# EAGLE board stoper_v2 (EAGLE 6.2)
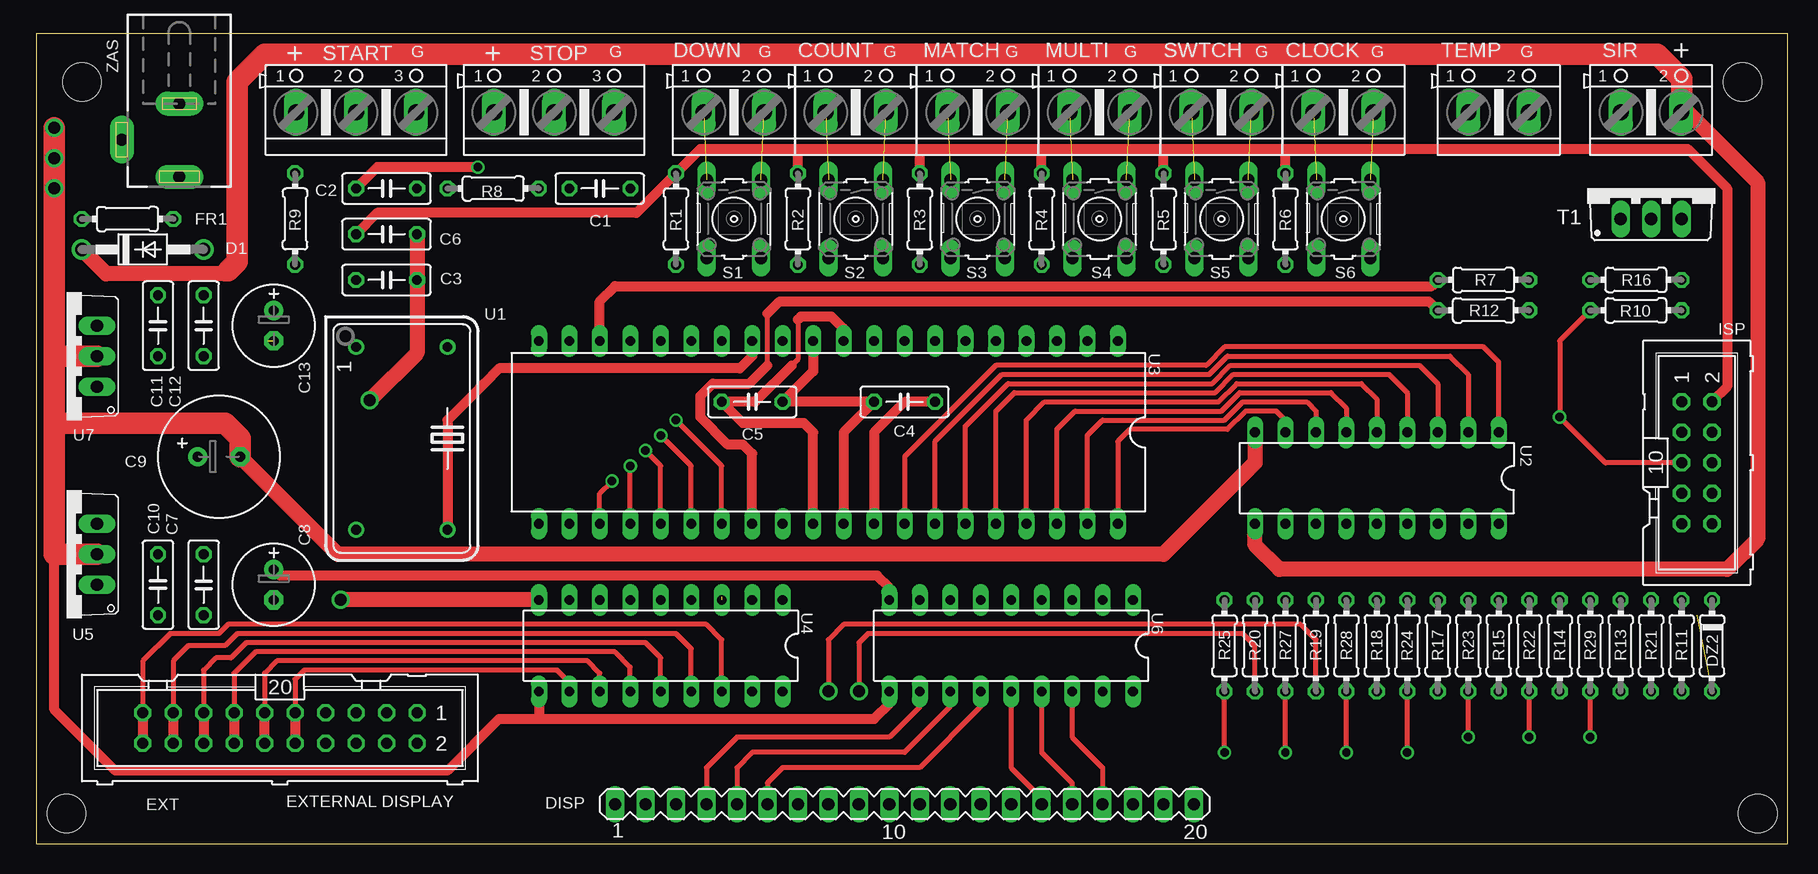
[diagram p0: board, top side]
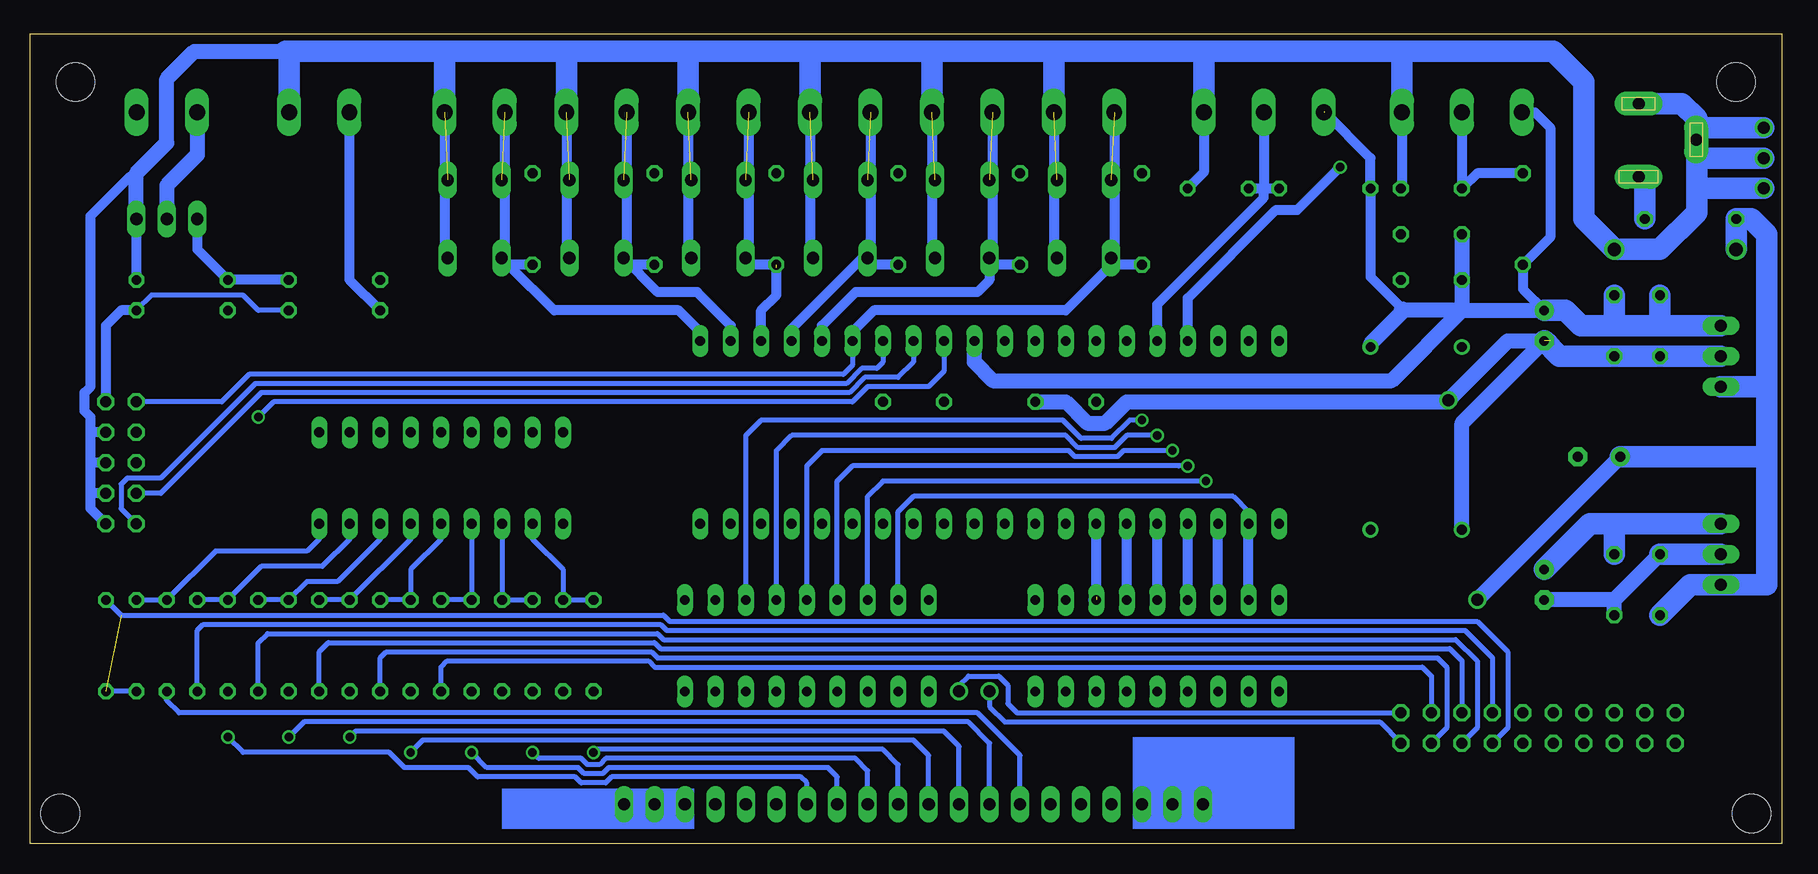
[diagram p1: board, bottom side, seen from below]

Size 146.03 x 67.49 mm. Coordinates in mm from the lower left corner, seen from the top.
Outline: 0,0 146.03,0 146.03,67.49 0,67.49 0,0
Copper layers (1*16): Top 0.035mm / dielectric 1.5mm / Bottom 0.035mm
Design rules: minimum track width 10mil, minimum drill 24mil, track to track 8mil, track to pad 8mil, pad to pad 8mil, via to via 8mil, smd to smd 8mil, copper to edge 40mil, drill to drill 8mil, minimum pad ring 10mil, minimum via ring 8mil, stop-mask expansion 4mil, vias tented up to drill 0mil, thermal gap 10mil
Holes 3.2 mm at 3.81,63.5 142.24,63.5 143.51,2.54 2.54,2.54

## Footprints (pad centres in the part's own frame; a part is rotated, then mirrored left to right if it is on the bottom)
AK500/2 = drill 1.321 long: 1 -2.515,0; 2 2.515,0
C050-025X075 = drill 0.813 octagon: 1 -2.54,0; 2 2.54,0
E2,5-7 = drill 0.813 pad 1.6: + -1.27,0 | drill 0.813 pad 1.6 octagon: - 1.27,0
E3,5-10 = drill 0.813 pad 1.6: + -1.778,0 | drill 0.813 pad 1.6 octagon: - 1.778,0
DO41-10 = drill 1.118: A 5.08,0; C -5.08,0
MA20-1 = drill 1.016 long: 1 -24.13,0; 2 -21.59,0; 3 -19.05,0; 4 -16.51,0; 5 -13.97,0; 6 -11.43,0; 7 -8.89,0; 8 -6.35,0; 9 -3.81,0; 10 -1.27,0; 11 1.27,0; 12 3.81,0; 13 6.35,0; 14 8.89,0; 15 11.43,0; 16 13.97,0; 17 16.51,0; 18 19.05,0; 19 21.59,0; 20 24.13,0
0204/7 = drill 0.813 octagon: 1 -3.81,0; 2 3.81,0
ML20 = drill 0.914 octagon: 1 -11.43,-1.27; 2 -11.43,1.27; 3 -8.89,-1.27; 4 -8.89,1.27; 5 -6.35,-1.27; 6 -6.35,1.27; 7 -3.81,-1.27; 8 -3.81,1.27; 9 -1.27,-1.27; 10 -1.27,1.27; 11 1.27,-1.27; 12 1.27,1.27; 13 3.81,-1.27; 14 3.81,1.27; 15 6.35,-1.27; 16 6.35,1.27; 17 8.89,-1.27; 18 8.89,1.27; 19 11.43,-1.27; 20 11.43,1.27
ML10 = drill 0.914 octagon: 1 -5.08,-1.27; 2 -5.08,1.27; 3 -2.54,-1.27; 4 -2.54,1.27; 5 0,-1.27; 6 0,1.27; 7 2.54,-1.27; 8 2.54,1.27; 9 5.08,-1.27; 10 5.08,1.27
B3F-10XX = drill 1.016 long: 1 -3.251,2.261; 2 3.251,2.261; 3 -3.251,-2.261; 4 3.251,-2.261
TO220BV = drill 1.016 long: D 0,-2.54; G -2.54,-2.54; S 2.54,-2.54
DIL14S = drill 0.813: 1 -7.62,-3.81; 7 7.62,-3.81; 8 7.62,3.81; 14 -7.62,3.81
DIL18 = drill 0.813 long: 1 -10.16,-3.81; 2 -7.62,-3.81; 3 -5.08,-3.81; 4 -2.54,-3.81; 5 0,-3.81; 6 2.54,-3.81; 7 5.08,-3.81; 8 7.62,-3.81; 9 10.16,-3.81; 10 10.16,3.81; 11 7.62,3.81; 12 5.08,3.81; 13 2.54,3.81; 14 0,3.81; 15 -2.54,3.81; 16 -5.08,3.81; 17 -7.62,3.81; 18 -10.16,3.81
DIL40 = drill 0.813 long: 1 -24.13,-7.62; 2 -21.59,-7.62; 3 -19.05,-7.62; 4 -16.51,-7.62; 5 -13.97,-7.62; 6 -11.43,-7.62; 7 -8.89,-7.62; 8 -6.35,-7.62; 9 -3.81,-7.62; 10 -1.27,-7.62; 11 1.27,-7.62; 12 3.81,-7.62; 13 6.35,-7.62; 14 8.89,-7.62; 15 11.43,-7.62; 16 13.97,-7.62; 17 16.51,-7.62; 18 19.05,-7.62; 19 21.59,-7.62; 20 24.13,-7.62; 21 24.13,7.62; 22 21.59,7.62; 23 19.05,7.62; 24 16.51,7.62; 25 13.97,7.62; 26 11.43,7.62; 27 8.89,7.62; 28 6.35,7.62; 29 3.81,7.62; 30 1.27,7.62; 31 -1.27,7.62; 32 -3.81,7.62; 33 -6.35,7.62; 34 -8.89,7.62; 35 -11.43,7.62; 36 -13.97,7.62; 37 -16.51,7.62; 38 -19.05,7.62; 39 -21.59,7.62; 40 -24.13,7.62
TO220V = drill 1.016 long: 1 -2.54,-2.54; 2 0,-2.54; 3 2.54,-2.54
AK500/3 = drill 1.321 long: 1 -5.004,0; 2 0,0; 3 5.004,0
DCJ0202 = drill 1 pad 2 long: 1 0,3.1; 2 4.8,0; 3 0,-3

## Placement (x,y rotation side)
1W  [AK500/2]  121.92,60.96 0 top
C1  100nF  [C050-025X075]  46.99,54.61 0 top
C2  100nF  [C050-025X075]  29.21,54.61 0 top
C3  100nF  [C050-025X075]  29.21,46.99 0 top
C4  100nF  [C050-025X075]  72.39,36.83 180 top
C5  100nF  [C050-025X075]  59.69,36.83 0 top
C6  100nF  [C050-025X075]  29.21,50.8 0 top
C7  100nF  [C050-025X075]  13.97,21.59 270 top
C8  100uF  [E2,5-7]  19.81,21.59 270 top
C9  1000/25  [E3,5-10]  15.24,32.26 0 top
C10  100nF  [C050-025X075]  10.16,21.59 90 top
C11  100nF  [C050-025X075]  10.16,43.18 270 top
C12  100nF  [C050-025X075]  13.97,43.18 270 top
C13  100uF  [E2,5-7]  19.81,43.18 270 top
D1  [DO41-10]  8.89,49.53 0 top
DISP  [MA20-1]  72.39,3.3 0 top
DOWN  [AK500/2]  108.97,60.96 0 top
DZ2  100  [0204/7]  139.7,16.51 270 top
EXT  [ML20]  20.32,9.65 180 top
FR1  [0204/7]  7.62,52.07 0 top
ISP  [ML10]  138.43,31.75 270 top
MODE  [AK500/2]  88.65,60.96 0 top
R1  10k  [0204/7]  53.34,52.07 270 top
R2  10k  [0204/7]  63.5,52.07 270 top
R3  10k  [0204/7]  73.66,52.07 270 top
R4  10k  [0204/7]  83.82,52.07 270 top
R5  10k  [0204/7]  93.98,52.07 270 top
R6  10k  [0204/7]  104.14,52.07 270 top
R7  2.2k  [0204/7]  120.65,44.45 0 top
R8  22k  [0204/7]  38.1,54.61 0 top
R9  22k  [0204/7]  21.59,52.07 90 top
R10  10k  [0204/7]  133.35,44.45 180 top
R11  100  [0204/7]  137.16,16.51 270 top
R12  2.2k  [0204/7]  120.65,46.99 180 top
R13  100  [0204/7]  132.08,16.51 270 top
R14  100  [0204/7]  127,16.51 270 top
R15  100  [0204/7]  121.92,16.51 270 top
R16  10k  [0204/7]  133.35,46.99 180 top
R17  100  [0204/7]  116.84,16.51 270 top
R18  100  [0204/7]  111.76,16.51 270 top
R19  100  [0204/7]  106.68,16.51 270 top
R20  100  [0204/7]  101.6,16.51 270 top
R21  100  [0204/7]  134.62,16.51 270 top
R22  100  [0204/7]  124.46,16.51 270 top
R23  100  [0204/7]  119.38,16.51 270 top
R24  100  [0204/7]  114.3,16.51 270 top
R25  100  [0204/7]  99.06,16.51 270 top
R27  100  [0204/7]  104.14,16.51 270 top
R28  100  [0204/7]  109.22,16.51 270 top
R29  100  [0204/7]  129.54,16.51 270 top
RESET  [AK500/2]  78.49,60.96 0 top
S1  [B3F-10XX]  58.17,52.07 270 top
S2  [B3F-10XX]  68.33,52.07 270 top
S3  [B3F-10XX]  78.49,52.07 270 top
S4  [B3F-10XX]  88.65,52.07 270 top
S5  [B3F-10XX]  98.81,52.07 270 top
S6  [B3F-10XX]  108.97,52.07 270 top
START  [AK500/2]  58.17,60.96 0 top
STOP  [AK500/2]  68.33,60.96 0 top
T1  IRF540  [TO220BV]  134.62,54.61 0 top
U1  10MHz  [DIL14S]  30.48,33.78 270 top
U2  ULN2803  [DIL18]  111.76,30.48 180 top
U3  ATmega16  [DIL40]  66.04,34.29 180 top
U4  UDN2983A  [DIL18]  52.07,16.51 180 top
U5  7808  [TO220V]  2.54,24.13 90 top
U6  UDN2983A  [DIL18]  81.28,16.51 180 top
U7  7805  [TO220V]  2.54,40.64 90 top
UP  [AK500/2]  98.81,60.96 0 top
X1  [AK500/3]  43.18,60.96 0 top
X2  [AK500/3]  26.67,60.96 0 top
X3  [AK500/2]  134.62,60.96 0 top
ZAS  [DCJ0202]  11.94,58.67 180 top

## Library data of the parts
1W DOWN MODE RESET START STOP UP X1-X3 = con-ptr500; OC_FARNELL: unknown; OC_NEWARK: unknown
C1-C13 DZ2 FR1 R1-R25 R27-R29 = rcl
D1 = diode
DISP = con-lstb; OC_FARNELL: unknown; OC_NEWARK: unknown
EXT ISP = con-harting-ml; OC_FARNELL: unknown; OC_NEWARK: unknown
S1-S6 = switch-omron; MPN: B3F-1000; OC_FARNELL: 176432; OC_NEWARK: 36M3542
T1 = transistor-power
U1 = crystal; OC_FARNELL: unknown; OC_NEWARK: unknown
U2 U4 U6 = uln-udn
U3 = atmel; MPN: ATMEGA16-16PU; OC_FARNELL: 9171142; OC_NEWARK: 01M6885
U5 U7 = linear
ZAS = con-jack; OC_FARNELL: unknown; OC_NEWARK: unknown

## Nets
1A: R20.1 R25.1 U2.11
1B: R19.1 R27.1 U2.12
1C: R18.1 R28.1 U2.13
1D: R17.1 R24.1 U2.14
1DP: R11.1 R21.1 U2.18
1E: R15.1 R23.1 U2.15
1F: R14.1 R22.1 U2.16
1G: R13.1 R29.1 U2.17
1W: 1W.1 R7.1 U3.28
1W1: DISP.17 U6.16
1W2: DISP.16 U6.15
1W3: DISP.15 U6.14
1W4: DISP.6 U6.13
1W5: DISP.5 U6.12
1W6: DISP.4 U6.11
2A: EXT.1 R20.2
2B: EXT.2 R19.2
2C: EXT.3 R18.2
2D: EXT.4 R17.2
2DP: DZ2.1 DZ2.2 EXT.8 R11.2
2E: EXT.5 R15.2
2F: EXT.6 R14.2
2G: EXT.7 R13.2
2W1: EXT.19 EXT.20 U4.16
2W2: EXT.17 EXT.18 U4.15
2W3: EXT.15 EXT.16 U4.14
2W4: EXT.13 EXT.14 U4.13
2W5: EXT.11 EXT.12 U4.12
2W6: EXT.9 EXT.10 U4.11
+5V: C3.1 C5.1 C6.1 C11.1 C12.1 C13.+ ISP.2 R1.1 R2.1 R3.1 R4.1 R5.1 R6.1 R7.2 R8.1 R9.1 R10.1 U1.14 U3.10 U3.30 U7.3 X1.1 X2.1
A1: U3.27 U4.3 U6.3
A2: U3.26 U4.4 U6.4
A3: U3.25 U4.5 U6.5
A4: U3.24 U4.6 U6.6
A5: U3.23 U4.7 U6.7
A6: U3.22 U4.8 U6.8
GND: 1W.2 C1.2 C2.2 C3.2 C4.2 C5.2 C6.2 C7.2 C8.- C9.- C10.2 C11.2 C12.2 C13.- D1.A DOWN.2 ISP.4 ISP.6 ISP.8 ISP.10 MODE.2 R16.1 RESET.2 S1.1 S1.2 S2.1 S2.2 S3.1 S3.2 S4.1 S4.2 S5.1 S5.2 S6.1 S6.2 START.2 STOP.2 T1.S U1.7 U2.9 U3.11 U3.31 U4.10 U5.2 U6.10 U7.2 UP.2 X1.3 X2.3 ZAS.2 ZAS.3
INT0: C1.1 R8.2 U3.16 X1.2
INT1: C2.1 R9.2 U3.17 X2.2
MISO: ISP.9 U3.7
N$1: U1.8 U3.13
N$2: C4.1 U3.32
N$3: R12.1 R16.2 T1.G
N$4: U2.1 U3.33
N$5: U2.2 U3.34
N$6: FR1.2 ZAS.1
N$7: U2.3 U3.35
N$8: U2.4 U3.36
N$9: U2.5 U3.37
N$10: U2.6 U3.38
N$11: U2.7 U3.39
N$12: U2.8 U3.40
N$13: T1.D X3.1
N$14: DISP.8 R22.2
N$15: DISP.7 R21.2
N$23: DISP.9 R23.2
N$24: DISP.10 R24.2
N$25: DISP.11 R25.2
N$26: DISP.12 R27.2
N$27: DISP.13 R28.2
N$28: DISP.14 R29.2
OUT: R12.2 U3.18
RST: ISP.5 R10.2 U3.9
S1: ISP.1 R1.2 S1.3 S1.4 START.1 U3.6
S2: R2.2 S2.3 S2.4 STOP.1 U3.5
S3: R3.2 RESET.1 S3.3 S3.4 U3.4
S4: MODE.1 R4.2 S4.3 S4.4 U3.3
S5: R5.2 S5.3 S5.4 U3.2 UP.1
S6: DOWN.1 R6.2 S6.3 S6.4 U3.1
SCK: ISP.7 U3.8
V+: C7.1 C8.+ U5.3 U6.9
VCC: C9.+ C10.1 D1.C FR1.1 U2.10 U4.9 U5.1 U7.1 X3.2

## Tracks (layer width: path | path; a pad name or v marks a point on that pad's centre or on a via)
1A
  Bottom 0.406: R25.1 R20.1 101.6,22.86 104.14,25.4 U2.11
1B
  Bottom 0.406: U2.12 R19.1 R27.1
1C
  Bottom 0.406: U2.13 R28.1 R18.1
1D
  Bottom 0.406: R17.1 R24.1 114.3,22.86 111.76,25.4 U2.14
1DP
  Bottom 0.406: U2.18 121.92,25.4 122.94,24.38 130.56,24.38 R21.1 R11.1
1E
  Bottom 0.406: U2.15 114.3,25.4 R23.1 R15.1
1F
  Bottom 0.406: U2.16 116.84,25.4 120.4,21.84 122.94,21.84 R22.1 R14.1
1G
  Bottom 0.406: U2.17 119.38,25.4 121.67,23.11 126.75,23.11 R29.1 R13.1
1W
  Top 0.406: 60.96,39.88 60.96,44.2
  Top 0.813: U3.28 59.69,32.51 58.93,33.27 57.66,33.27 55.37,35.56 55.37,37.34 56.39,38.35 59.44,38.35 60.96,39.88 | 60.96,44.2 61.98,45.21 116.08,45.21 R7.1
  Bottom 0.813: 1W.1 119.41,47.02 R7.1
1W1
  Top 0.406: U6.16 86.36,8.89 88.9,6.35 DISP.17
1W2
  Top 0.406: U6.15 83.82,7.62 86.36,5.08 DISP.16
1W3
  Top 0.406: U6.14 81.28,6.35 83.82,3.81 DISP.15
1W4
  Top 0.406: U6.13 78.74,11.43 73.66,6.35 62.23,6.35 60.96,5.08 DISP.6
1W5
  Top 0.406: U6.12 76.2,11.43 72.39,7.62 59.69,7.62 58.42,6.35 DISP.5
1W6
  Top 0.406: U6.11 73.66,11.43 71.12,8.89 58.42,8.89 55.88,6.35 DISP.4
2A  (via drill 1)
  Top 0.406: R20.2 101.6,16.51 100.58,17.53 69.34,17.53 68.58,16.76 v68.58,12.7
  Bottom 0.406: v68.58,12.7 68.58,13.21 67.82,13.97 65.28,13.97 64.52,13.21 64.52,11.68 63.75,10.92 EXT.1
2B  (via drill 1)
  Top 0.406: R19.2 106.68,17.02 105.41,18.29 67.31,18.29 66.04,17.02 v66.04,12.7
  Bottom 0.406: v66.04,12.7 66.04,11.43 64.77,10.16 33.53,10.16 EXT.2
2C
  Bottom 0.406: R18.2 111.76,14.73 111.25,15.24 94.49,15.24 93.98,14.73 29.97,14.73 29.21,13.97 EXT.3
2D
  Bottom 0.406: R17.2 116.84,15.49 116.33,16 94.23,16 93.73,15.49 28.7,15.49 27.94,14.73 27.94,9.65 EXT.4
2DP  (1 unrouted)
  Bottom 0.406: DZ2.1 138.43,19.05 93.22,19.05 92.71,18.54 25.4,18.54 22.86,16 22.86,9.65 EXT.8 | R11.2 DZ2.2
2E
  Bottom 0.406: R15.2 121.92,16 121.16,16.76 93.98,16.76 93.47,16.26 27.69,16.26 26.67,15.24 EXT.5
2F
  Bottom 0.406: R14.2 127,16.76 126.24,17.53 93.73,17.53 93.22,17.02 27.18,17.02 25.4,15.24 25.4,9.65 EXT.6
2G
  Bottom 0.406: R13.2 132.08,17.78 131.57,18.29 93.47,18.29 92.96,17.78 26.42,17.78 24.13,15.49 EXT.7
2W1
  Top 0.406: U4.16 57.15,17.02 55.88,18.29 16,18.29 15.24,17.53 11.18,17.53 8.89,15.24 EXT.19
  Top 0.813: EXT.19 EXT.20
2W2
  Top 0.406: U4.15 54.61,16.26 53.34,17.53 16.76,17.53 15.75,16.51 12.7,16.51 11.43,15.24 EXT.17
  Top 0.813: EXT.17 EXT.18
2W3
  Top 0.406: U4.14 52.07,15.49 50.8,16.76 17.53,16.76 16.26,15.49 14.99,15.49 13.97,14.48 EXT.15
  Top 0.813: EXT.15 EXT.16
2W4
  Top 0.406: U4.13 49.53,14.73 48.26,16 18.29,16 16.51,14.22 EXT.13
  Top 0.813: EXT.13 EXT.14
2W5
  Top 0.406: U4.12 46.99,14.22 45.97,15.24 20.07,15.24 19.05,14.22 EXT.11
  Top 0.813: EXT.12 EXT.11
2W6
  Top 0.406: U4.11 44.45,13.46 43.43,14.48 22.35,14.48 21.59,13.72 EXT.9
  Top 0.813: EXT.9 EXT.10
+5V  (1 unrouted)
  Top 0.406: 63.5,43.69 63.5,40.39 62.99,39.88
  Top 0.813: 63.5,57.91 55.37,57.91 R1.1 50.04,52.58 28.45,52.58 C6.1 | 63.5,57.91 73.66,57.91 | 73.66,57.91 83.82,57.91 | 83.82,57.91 93.98,57.91 | R5.1 93.98,57.91 | R4.1 83.82,57.91 | R3.1 73.66,57.91 | R2.1 63.5,57.91 | U3.30 64.77,34.29 64.01,35.05 58.93,35.05 C5.1 59.94,36.83 62.99,39.88 | U3.10 67.31,42.93 66.29,43.94 63.75,43.94 63.5,43.69 | 93.98,57.91 104.14,57.91 | 104.14,57.91 137.67,57.91 140.97,54.61 140.97,38.1 ISP.2 | R6.1 104.14,57.91
  Bottom 0.406: R7.2 127,44.45 128.27,45.72 135.89,45.72 R10.1
  Bottom 0.813: X2.1 20.57,60.96 19.3,59.69 19.3,50.55 R9.1 21.59,46.23 C13.+ | 38.1,60.96 34.29,57.15 R8.1 34.29,47.24 31.62,44.58 | ISP.2 139.7,43.18 138.43,44.45 R10.1
  Bottom 1.27: 26.67,44.45 31.5,44.45 | 31.5,44.45 31.75,44.45 31.62,44.58 | 26.67,44.45 C3.1 C6.1 | 26.67,44.45 19.3,44.45 | 26.67,44.45 32.51,38.61 65.79,38.61 67.31,40.13 U3.10 | U1.14 34.29,41.66 31.5,44.45
  Bottom 1.778: U7.3 9.91,43.18 | 9.91,43.18 13.97,43.18 | 13.97,43.18 16.76,43.18 18.03,44.45 19.3,44.45 C13.+ | C12.1 13.97,43.18 | C11.1 10.16,43.43 9.91,43.18
A1  (via drill 0.7)  (1 unrouted)
  Top 0.406: U3.27 57.15,31.5 v53.34,35.31
  Bottom 0.406: U6.3 86.36,34.04 85.09,35.31 59.94,35.31 58.42,33.78 55.88,33.78 54.36,35.31 v53.34,35.31
  Bottom 0.813: 57.4,20.32 57.15,20.57 U3.27
A2  (via drill 0.7)
  Top 0.406: U3.26 54.61,31.5 v52.07,34.04
  Bottom 0.406: v52.07,34.04 54.61,34.04 55.63,33.02 58.67,33.02 59.69,34.04 82.55,34.04 83.82,32.77 U6.4
  Bottom 0.813: U4.4 U3.26
A3  (via drill 0.7)
  Top 0.406: U3.25 52.07,31.5 v50.8,32.77
  Bottom 0.406: v50.8,32.77 54.86,32.77 55.37,32.26 58.93,32.26 59.44,32.77 80.01,32.77 81.28,31.5 U6.5
  Bottom 0.813: U4.5 U3.25
A4  (via drill 0.7)
  Top 0.406: U3.24 v49.53,31.5
  Bottom 0.406: U6.6 78.74,30.23 77.47,31.5 50.29,31.5 v49.53,31.5
  Bottom 0.813: U4.6 U3.24
A5  (via drill 0.7)
  Top 0.406: U3.23 46.99,29.21 v48.01,30.23
  Bottom 0.406: v48.01,30.23 74.93,30.23 76.2,28.96 U6.7
  Bottom 0.813: U4.7 U3.23
A6
  Bottom 0.406: U6.8 73.66,27.69 72.39,28.96 45.72,28.96 44.45,27.69 U3.22
  Bottom 0.813: U4.8 U3.22
GND  (via drill 1)  (7 unrouted)
  Top 0.813: U3.31 67.31,34.29 C4.2 C5.2 64.77,39.37 U3.11 | 42.16,10.41 38.61,10.41 34.29,6.1 6.6,6.1 1.52,11.18 1.52,24.13 | 42.16,10.41 69.85,10.41 71.12,11.68 U6.10 | U4.10 41.91,10.67 42.16,10.41
  Top 1.27: C6.2 C3.2 31.75,40.89 v27.81,36.96 | U2.9 101.6,31.75 93.98,24.13 25.15,24.13 C9.-
  Top 1.778: C9.- 17.02,33.78 15.75,35.05 1.78,35.05 | 1.78,35.05 1.52,35.05 1.52,40.64 | U7.2 1.52,40.64 | U5.2 1.52,24.13 1.52,34.8 1.78,35.05 | 1.52,40.64 v1.52,54.61 v1.52,57.15 v1.52,59.69
  Bottom 0.813: X1.3 48.18,55.96 C1.2 | START.2 60.68,49.07 S1.2 | STOP.2 70.84,49.07 S2.2 | RESET.2 81,49.07 S3.2 | MODE.2 91.16,49.07 S4.2 | UP.2 101.32,49.07 S5.2 | X2.3 31.67,54.69 C2.2 | ISP.10 140.97,27.94 140.97,29.21 | 140.97,29.21 140.97,31.5 | 140.97,31.5 140.97,34.29 | 140.97,34.29 140.97,35.56 141.48,36.07 141.48,37.59 140.97,38.1 140.97,52.32 137.67,55.63 137.41,55.63 137.16,55.88 | ISP.4 140.97,34.29 | ISP.6 140.72,31.75 140.97,31.5 | ISP.8 140.97,29.21 | T1.S R16.1 | DOWN.2 111.48,49.07 S6.2
  Bottom 1.27: U1.7 26.67,35.05 C13.- | C5.2 59.69,36.83 57.91,35.05 56.39,35.05 54.61,36.83 27.94,36.83 v27.81,36.96 22.86,41.91 19.3,41.91 | C10.2 13.97,20.32 | 13.97,20.32 C8.- | C7.2 13.97,20.32 | T1.S 137.16,55.88 134.62,58.42 134.62,63.75 132.33,66.04 124.71,66.04 124.47,66.04 124.33,65.91
  Bottom 1.778: U7.2 C11.2 C12.2 18.54,40.64 C13.- | 7.11,57.15 7.11,52.58 10.16,49.53 D1.A 16.51,52.07 16.51,63.5 19.05,66.04 31.75,66.04 | 7.11,57.15 7.11,58.65 | 7.11,58.65 ZAS.2 7.11,58.7 | ZAS.3 8.33,61.67 7.11,60.45 7.11,59.69 | 7.11,59.69 7.11,58.7 | U5.2 C10.2 | X2.3 31.67,65.96 31.75,66.04 | 1W.2 124.44,65.76 124.71,66.04 111.25,66.04 | 111.25,66.04 101.35,66.04 | 101.35,66.04 90.93,66.04 | 90.93,66.04 80.77,66.04 | 80.77,66.04 70.87,66.04 | 70.87,66.04 60.45,66.04 | 60.45,66.04 48.26,66.04 | 48.26,66.04 31.75,66.04 | X1.3 48.18,65.96 48.26,66.04 | START.2 60.68,65.81 60.45,66.04 | STOP.2 70.84,66.02 70.87,66.04 | RESET.2 81,65.81 80.77,66.04 | MODE.2 91.16,65.81 90.93,66.04 | UP.2 101.32,66.02 101.35,66.04 | DOWN.2 111.48,65.81 111.25,66.04 | v1.52,59.69 7.11,59.69 | 7.11,58.7 7.11,58.65 | 7.11,57.15 v1.52,57.15 | v1.52,54.61 6.86,54.61
INT0
  Bottom 0.813: C1.1 43.18,54.61 | 43.18,54.61 R8.2 | X1.2 43.18,54.61 | U3.16 52.07,44.96 43.18,53.85 43.18,54.61
INT1  (via drill 0.7)
  Top 0.813: v36.83,56.39 28.45,56.39 C2.1
  Bottom 0.813: X2.2 C2.1 25.4,55.88 R9.2 | U3.17 49.53,45.47 42.16,52.83 40.39,52.83 v36.83,56.39
MISO
  Bottom 0.406: U3.7 74.93,40.13 75.44,39.62 76.71,39.62 77.98,38.35 127.25,38.35 135.13,30.48 137.92,30.48 138.43,29.97 138.43,27.94 ISP.9
N$1
  Top 0.813: U1.8 34.29,35.31 36.96,37.97 37.34,38.35 38.61,39.62 58.67,39.62 59.69,40.64 U3.13
N$2
  Top 0.813: C4.1 72.39,36.83 69.85,34.29 U3.32
N$3
  Bottom 0.813: R12.1 R16.2 132.08,49.53 T1.G
N$4
  Top 0.406: U2.1 121.92,40.13 120.65,41.4 99.06,41.4 97.54,39.88 80.01,39.88 72.39,32.26 U3.33
N$5
  Top 0.406: U3.34 74.93,33.53 80.52,39.12 97.79,39.12 99.31,40.64 117.86,40.64 119.38,39.12 U2.2
N$6
  Bottom 1.778: ZAS.1 11.43,55.57 FR1.2
N$7
  Top 0.406: U3.35 77.47,34.8 81.03,38.35 98.04,38.35 99.57,39.88 115.32,39.88 116.84,38.35 U2.3
N$8
  Top 0.406: U3.36 80.01,36.07 81.53,37.59 98.3,37.59 99.82,39.12 112.78,39.12 114.3,37.59 U2.4
N$9
  Top 0.406: U3.37 82.55,35.31 84.07,36.83 98.55,36.83 100.08,38.35 110.49,38.35 111.76,37.08 U2.5
N$10
  Top 0.406: U3.38 85.09,34.54 86.61,36.07 98.81,36.07 100.33,37.59 107.95,37.59 109.22,36.32 U2.6
N$11
  Top 0.406: U3.39 87.63,34.04 88.9,35.31 99.06,35.31 100.58,36.83 105.92,36.83 106.68,36.07 U2.7
N$12
  Top 0.406: U2.8 104.14,35.31 103.38,36.07 100.84,36.07 99.31,34.54 91.19,34.54 90.17,33.53 U3.40
N$13
  Bottom 1.27: X3.1 132.1,60.73 132.08,60.71 132.08,57.4 134.62,54.86 T1.D
N$14  (via drill 0.7)
  Top 0.406: v124.46,8.89 R22.2
  Bottom 0.406: DISP.8 66.04,8.38 67.82,10.16 123.19,10.16 v124.46,8.89
N$15
  Bottom 0.406: DISP.7 63.5,7.37 67.06,10.92 133.6,10.92 134.62,11.94 R21.2
N$23  (via drill 0.7)
  Top 0.406: v119.38,8.89 R23.2
  Bottom 0.406: DISP.9 68.58,8.13 69.85,9.4 118.87,9.4 v119.38,8.89
N$24  (via drill 0.7)
  Top 0.406: v114.3,7.62 R24.2
  Bottom 0.406: DISP.10 71.12,7.37 72.39,8.64 113.28,8.64 v114.3,7.62
N$25  (via drill 0.7)
  Top 0.406: v99.06,7.62 R25.2
  Bottom 0.406: DISP.11 73.66,6.6 74.93,7.87 98.81,7.87 v99.06,7.62
N$26  (via drill 0.7)
  Top 0.406: v104.14,7.62 R27.2
  Bottom 0.406: DISP.12 76.2,6.1 77.22,7.11 98.04,7.11 98.55,6.6 99.57,6.6 100.08,7.11 103.63,7.11 v104.14,7.62
N$27  (via drill 0.7)
  Top 0.406: v109.22,7.62 R28.2
  Bottom 0.406: DISP.13 78.74,5.59 79.5,6.35 97.79,6.35 98.3,5.84 99.82,5.84 100.33,6.35 107.95,6.35 v109.22,7.62
N$28  (via drill 0.7)
  Top 0.406: v129.54,8.89 R29.2
  Bottom 0.406: DISP.14 81.28,5.08 81.79,5.59 97.54,5.59 98.04,5.08 100.08,5.08 100.58,5.59 108.71,5.59 109.47,6.35 114.81,6.35 116.08,7.62 128.27,7.62 v129.54,8.89
OUT
  Top 0.813: U3.18 46.99,45.21 48.26,46.48 116.33,46.48 R12.2
RST  (via drill 0.7)
  Top 0.406: ISP.5 130.81,31.75 v127,35.56 127,41.91 R10.2
  Bottom 0.406: U3.9 69.85,39.37 71.12,38.1 76.2,38.1 77.47,36.83 125.73,36.83 v127,35.56
S1  (1 unrouted)
  Bottom 0.406: U3.6 77.47,39.88 78.23,39.12 127.76,39.12 130.05,36.83 ISP.1
  Bottom 0.813: START.1 55.65,49.07 S1.4 | R1.2 55.35,48.26 S1.4 | S1.4 55.91,48.23 59.69,44.45 75.69,44.45 77.47,42.67 U3.6
S2  (1 unrouted)
  Bottom 0.813: STOP.1 65.81,49.07 S2.4 | R2.2 65.51,48.26 S2.4 | S2.4 66.06,46.97 67.06,45.97 77.22,45.97 80.01,43.18 U3.5
S3  (1 unrouted)
  Bottom 0.813: RESET.1 75.97,49.07 S3.4 | R3.2 75.67,48.26 S3.4 | S3.4 76.22,48.74 76.73,48.74 82.55,42.93 82.55,42.16 U3.4 82.55,41.66
S4  (2 unrouted)
  Bottom 0.813: MODE.1 86.13,49.07 S4.4 85.83,48.26 R4.2 | U3.3 85.09,44.45 83.82,45.72 83.82,48.01 83.57,48.26
S5  (1 unrouted)
  Bottom 0.813: UP.1 96.29,49.07 S5.4 | R5.2 95.99,48.26 S5.4 | U3.2 87.63,43.18 90.42,45.97 93.7,45.97 S5.4
S6  (1 unrouted)
  Bottom 0.813: DOWN.1 106.45,49.07 S6.4 106.03,48.15 | U3.1 90.17,42.67 91.95,44.45 102.34,44.45 106.03,48.15 | R6.2 105.92,48.26 106.03,48.15
SCK
  Bottom 0.406: U3.8 72.39,40.13 73.66,38.86 76.45,38.86 77.72,37.59 126.75,37.59 135.13,29.21 ISP.7
V+
  Top 0.813: U6.9 71.12,21.34 70.1,22.35 20.32,22.35 C8.+
  Bottom 1.778: U5.3 13.97,26.67 | 13.97,26.67 16,26.67 C8.+ | C7.1 13.97,26.67
VCC  (via drill 1)
  Top 1.27: 16,47.75 15.75,47.5 5.84,47.5 D1.C | U4.9 v25.4,20.32 | 137.16,61.47 137.29,61.34 | 137.29,61.34 143.51,55.12 143.51,25.4 140.97,22.86 103.63,22.86 101.6,24.89 U2.10 | X3.2 137.13,61.19 137.29,61.34
  Top 1.778: 16,47.75 16.76,48.51 16.76,63.5 19.05,65.79 135.13,65.79 137.16,63.75 137.16,61.47
  Bottom 1.27: v25.4,20.32 C9.+
  Bottom 1.778: 1.27,38.35 1.27,50.8 2.54,52.07 FR1.1 D1.C | 1.27,38.35 1.27,32.26 | 1.27,32.26 1.27,21.59 U5.1 7.62,21.59 C10.1 | C9.+ 1.27,32.26 | U7.1 1.52,38.1 1.27,38.35
(copper drawn outside any net)
  shapes: Bottom area x2

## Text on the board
tPlace: G | G | DOWN | G | COUNT | G | MATCH | G | MULTI | G | SWTCH | G | CLOCK | G | TEMP | G | SIR | + | START | + | STOP | + | DZ2 | EXTERNAL DISPLAY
